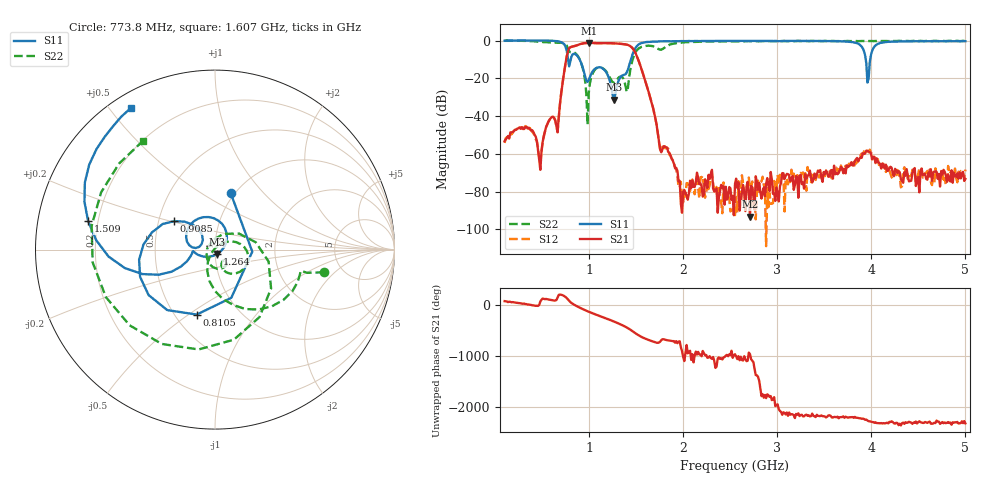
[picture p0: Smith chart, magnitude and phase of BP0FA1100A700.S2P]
! s2p File.  Ports: 1,3
# MHz S DB R 50
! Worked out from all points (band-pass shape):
!   401 points, 100 MHz to 5 GHz, reference 50 ohm
!   highest |S21| = -1.22 dB at 994.2 MHz (marker M1); lowest = -93.2 dB at 2.709 GHz (marker M2)
!   |S21| within 3 dB of the highest: 785.5 MHz to 1.463 GHz (677.9 MHz wide, 60.3 % of centre)
!   lowest |S11| = -31.2 dB at 1.264 GHz (marker M3), VSWR 1.06, Z = 51.2 - j2.52 ohm
!   |S11| at or under -10 dB: 774.7 MHz to 803 MHz (28.32 MHz wide, 3.59 % of centre); 898.1 MHz to 1.443 GHz (545.1 MHz wide, 46.6 % of centre); 3.94 GHz to 3.988 GHz (47.61 MHz wide, 1.2 % of centre)
!   |S22| runs from -44.5 to 0.0 dB; largest |S21 - S12| = 0.0041
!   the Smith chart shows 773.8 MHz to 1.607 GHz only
!   S11 on the Smith chart (normalised r, x): 773.8 MHz: 0.96, +0.68; 810.5 MHz: 0.64, -0.54; 908.5 MHz: 0.60, +0.21; 1.264 GHz: 1.02, -0.05; 1.509 GHz: 0.16, +0.11; 1.607 GHz: 0.06, +0.57
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100  -0.03 -12.8  -53.27 67.3  -54.22 65.8  -0.04 -33.4
479.75  0.06 -73.5  -68.47 59.5  -65.18 77.8  -0.52 169.5
639  -0.25 -120.8  -42.38 79.4  -42.21 80.7  -1.09 83.1
773.75  -9.70 74.5  -5.64 99.3  -5.66 99.3  -4.14 -11.8
810.5  -8.50 -105.7  -3.29 32.0  -3.27 31.8  -6.15 -15.9
908.5  -11.15 145.2  -1.78 -68.6  -1.79 -68.6  -11.10 -81.0
920.75  -12.77 137.4  -1.63 -79.3  -1.63 -79.2  -12.80 -90.4
994.25  -20.95 170.4  -1.22 -139.5  -1.23 -139.5  -27.96 46.8
1153.5  -15.13 92.3  -1.36 108.8  -1.37 108.8  -15.01 -47.6
1263.75  -31.25 -63.7  -1.42 29.6  -1.42 29.6  -22.31 -52.3
1398.5  -16.89 -164.0  -2.13 -85.7  -2.14 -85.7  -27.15 173.0
1508.75  -2.81 167.5  -8.55 140.4  -8.51 140.3  -4.98 -99.3
1606.75  -0.74 120.7  -23.12 48.4  -23.15 48.5  -2.78 123.7
1741.5  -0.41 89.0  -52.92 -18.9  -53.83 -21.2  -4.60 -64.5
1815  -0.34 77.7  -56.56 32.7  -57.04 26.3  -3.26 162.8
1925.25  -0.30 64.1  -67.43 7.3  -68.38 23.1  -1.32 79.9
2550  -0.14 26.9  -75.93 113.3  -92.44 -75.6  -0.35 -37.0
2709.25  -0.14 21.0  -93.25 115.1  -78.39 68.4  -0.34 -51.4
3370.75  -0.16 1.2  -75.20 37.4  -70.25 7.1  -0.20 -95.8
3958.75  -22.23 -88.8  -58.33 -98.7  -58.49 -90.3  -0.19 -123.8
4191.5  -0.61 1.5  -67.42 -124.6  -68.74 -133.5  -0.21 -133.2
5000  -0.30 -38.6  -73.31 -153.5  -68.34 -163.8  -0.14 -159.7
